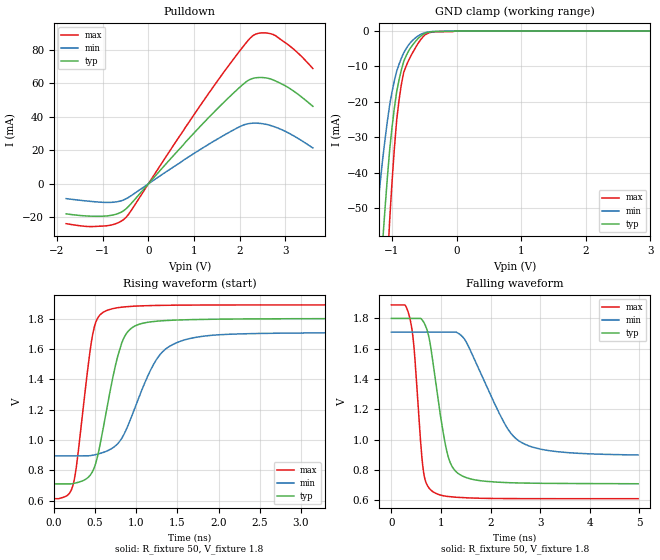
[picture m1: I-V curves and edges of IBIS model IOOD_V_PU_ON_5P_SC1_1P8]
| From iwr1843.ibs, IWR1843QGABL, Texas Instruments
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|   Model Cell IOOD_V_PU_ON_5P_SC1_1P8
|IOOD_V_PU_ON_5P_SC1_1P8
[Model]   IOOD_V_PU_ON_5P_SC1_1P8
Model_type   I/O_open_drain
Polarity   Non-Inverting
Enable   Active-Low
Vinl =  0.63
Vinh =  1.17
Cref =  15pF
Rref =  100.0000M
Vref =  0V
Vmeas =  0.9
|   typ   min   max
C_comp   2.233931p   2.204415p   2.290246p
[Model Spec]
Vinl   0.63   0.5985   0.6615
Vinh   1.17   1.1115   1.2285
[Temperature Range]   25   125   -40
[Voltage Range]   1.8   1.71   1.89
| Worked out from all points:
|   slope of the pulldown table from 0 to 0.27 V, typ, clamps not added: 32.2 ohm
|   GND clamp passes 1 mA (typ) near -0.52 V on its own axis
|   rising waveform, R_fixture 50, V_fixture 1.8: 20-80 % time 245ps typ, 395ps min, 168ps max; typ from 0.711 V to 1.8 V
|   falling waveform, R_fixture 50, V_fixture 1.8: 20-80 % time 308ps typ, 718ps min, 171ps max; typ from 1.8 V to 0.71 V
| Where Nom  PVT is Nominal Process, 1.8V, 25C
|   Fast PVT is Strong Process,  1.89V, -40C
|   Slow PVT is Weak Process,   1.71V, 125C
[Pulldown]
|   voltage   I(typ)   I(min)   I(max)
-1.8V     -17.92mA   -8.85mA    -23.8mA
-1.309V   -19.26mA   -10.37mA   -25.51mA
-927.3mV  -19.22mA   -11.12mA   -25.08mA
-654.5mV  -17.65mA   -10.56mA   -23.13mA
-490.9mV  -14.97mA   -8.985mA   -20.05mA
1.364V    40.78mA    24.32mA    55.7mA
2.073V    59.41mA    35mA       81.9mA
2.291V    62.96mA    36.2mA     88.48mA
2.509V    63.41mA    35.84mA    90.12mA
2.782V    61.38mA    33.82mA    88.42mA
3.218V    54.59mA    28.02mA    79.45mA
3.6V      46.26mA    21.39mA    68.79mA
[GND_clamp]
|   voltage   I(typ)   I(min)   I(max)
-1.8V     -270.2mA   -170.2mA   -430.1mA
-1.255V   -91.68mA   -55.92mA   -148.5mA
-1.145V   -59.94mA   -36.46mA   -97.14mA
-1.109V   -50.51mA   -30.84mA   -81.61mA
-1.073V   -41.77mA   -25.67mA   -67.13mA
-1.036V   -33.71mA   -20.95mA   -53.68mA
-927.3mV  -17.15mA   -11.38mA   -25.19mA
-854.5mV  -10.96mA   -7.663mA   -15.08mA
-781.8mV  -7.031mA   -5.001mA   -9.947mA
-563.6mV  -1.569mA   -1.041mA   -2.641mA
-18.18mV  0A         0A         0A
3.6V      0A         0A         0A
[Ramp]
| variable   typ   min   max
dV/dt_f 0.66095896/0.3106084n 0.49613312/0.73326127n 0.77259659/0.17250259n
dV/dt_r 0.65862655/0.43190461n 0.50230725/0.96092972n 0.77696157/0.24571965n
R_load = 50
[Rising Waveform]
R_fixture = 50
V_fixture = 1.8
V_fixture_min = 1.71
V_fixture_max = 1.89
|   time   V(typ)   V(min)   V(max)
0s        710.6mV    895.2mV    613.1mV
234.7ps   712.8mV    895.2mV    706mV
279.7ps   718.7mV    895.2mV    848.3mV
472.8ps   795.2mV    899.6mV    1.7V
625.3ps   1.154V     923mV      1.849V
773.2ps   1.547V     974.1mV    1.871V
891.9ps   1.709V     1.084V     1.879V
1.246ns   1.783V     1.53V      1.887V
1.553ns   1.791V     1.654V     1.889V
4.974ns   1.8V       1.708V     1.89V
[Falling Waveform]
R_fixture = 50
V_fixture = 1.8
V_fixture_min = 1.71
V_fixture_max = 1.89
|   time   V(typ)   V(min)   V(max)
0s        1.8V       1.71V      1.889V
275ps     1.8V       1.71V      1.889V
378.3ps   1.8V       1.71V      1.793V
458.3ps   1.8V       1.71V      1.601V
639.6ps   1.782V     1.71V      809mV
817.4ps   1.559V     1.71V      662.6mV
1.117ns   924.9mV    1.71V      627.2mV
1.374ns   771.8mV    1.697V     619.7mV
2.563ns   715.4mV    994.7mV    612.1mV
4.974ns   710.1mV    900mV      611.7mV
